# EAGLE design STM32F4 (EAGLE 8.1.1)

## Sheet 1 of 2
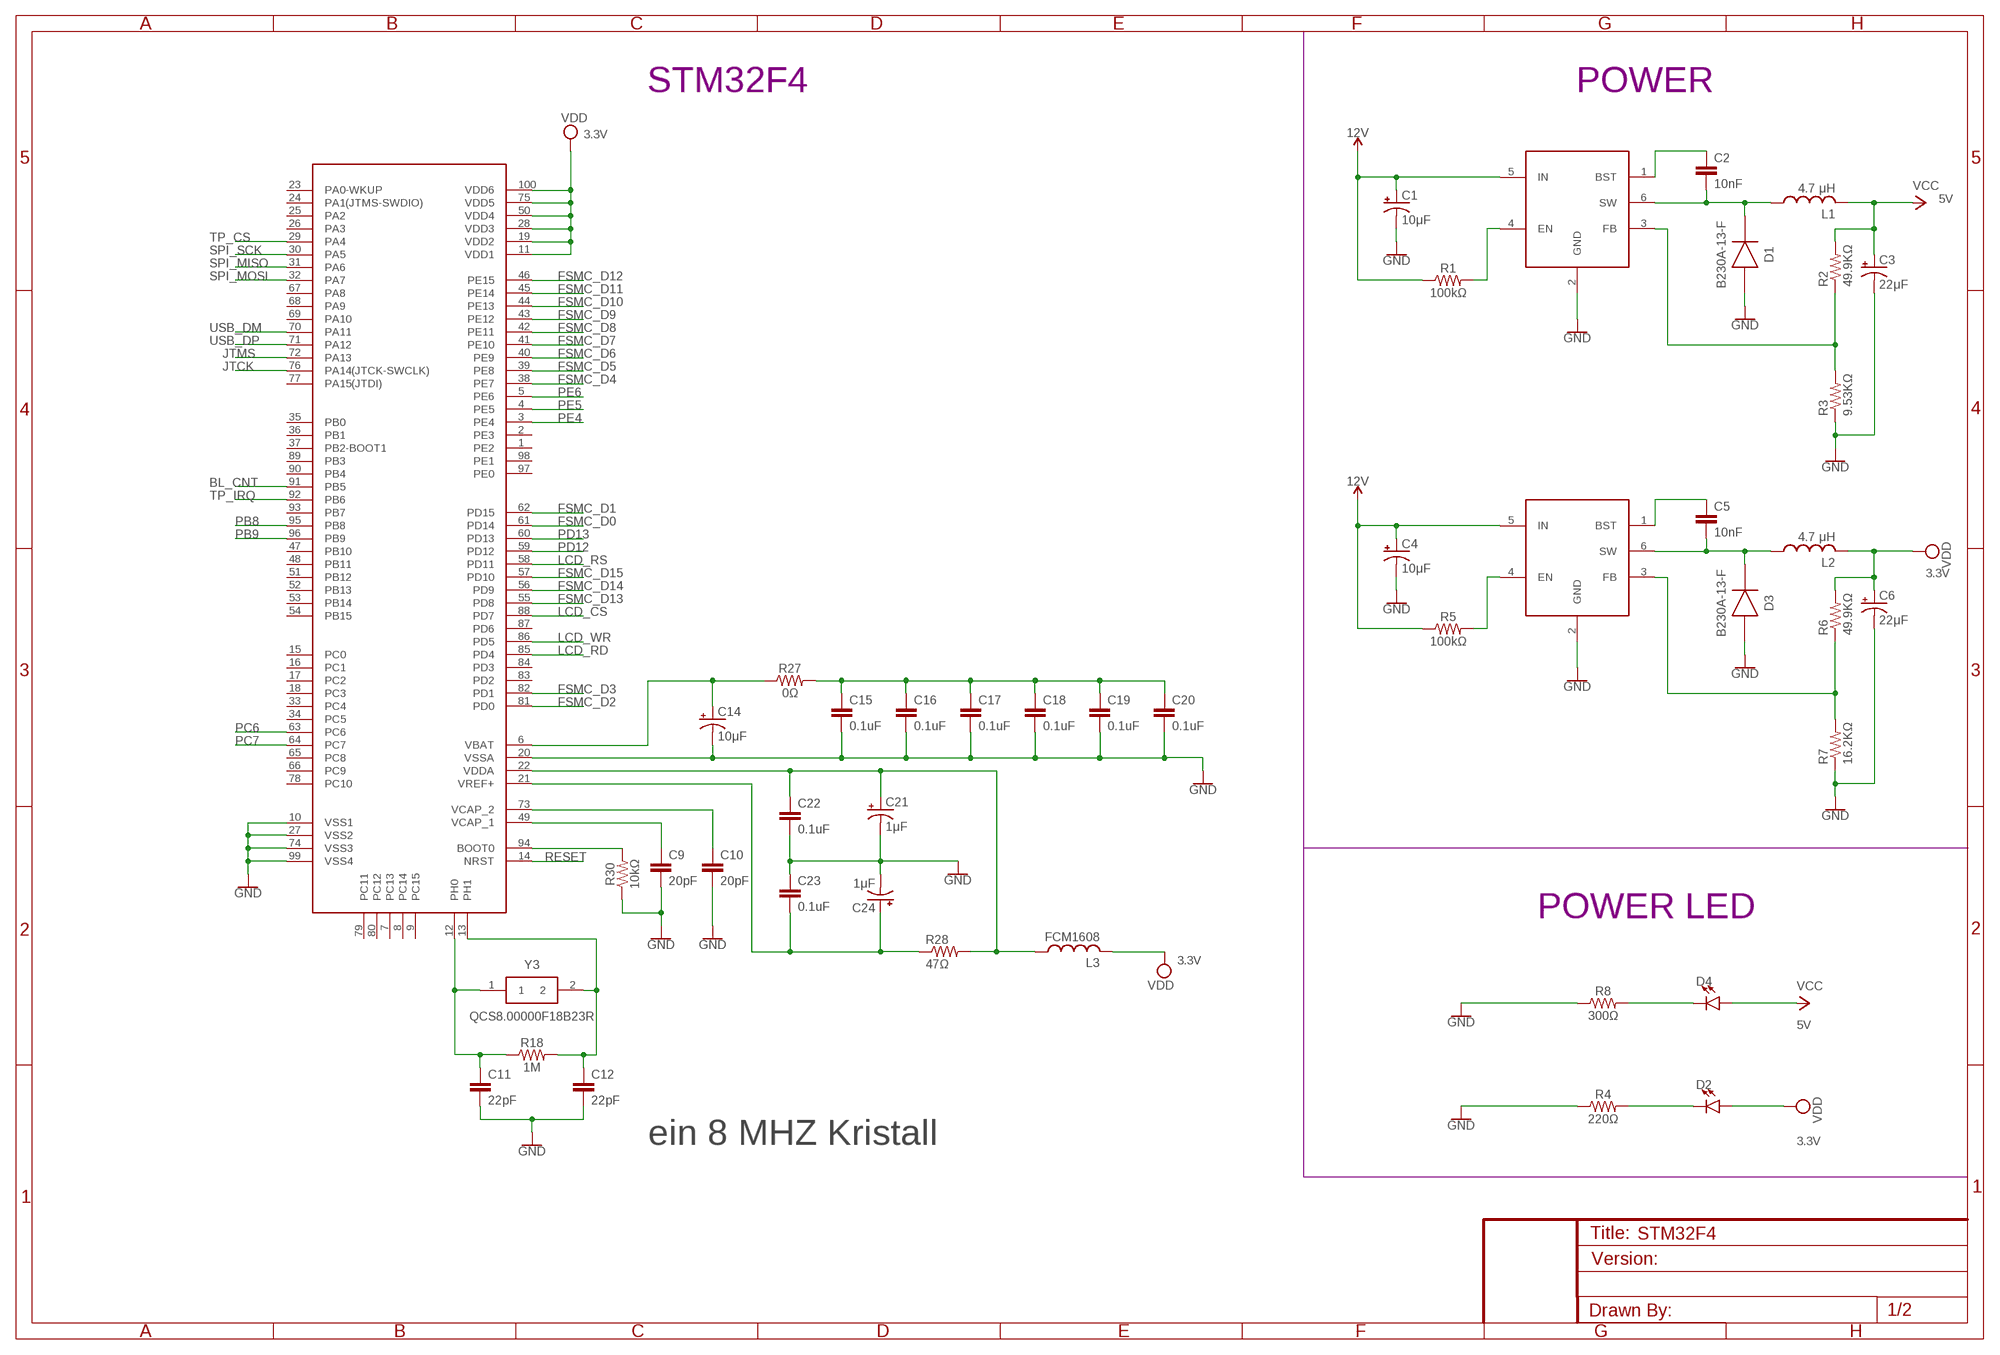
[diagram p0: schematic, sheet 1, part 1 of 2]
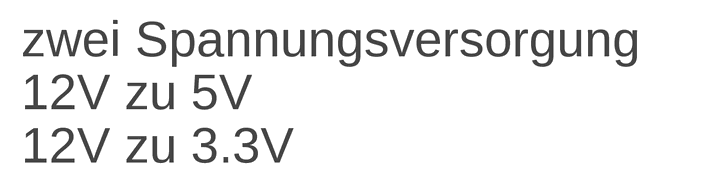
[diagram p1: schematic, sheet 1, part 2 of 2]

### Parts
C1  CAPACITOR_10UF  [E.CAPACITOR_10UF]
C2  10nF  10NF-0603-50V-10%  [0603]
C3  CAPACITOR_22UF  [E.CAPACITOR_10UF]
C4  CAPACITOR_10UF  [E.CAPACITOR_10UF]
C5  10nF  10NF-0603-50V-10%  [0603]
C6  CAPACITOR_22UF  [E.CAPACITOR_10UF]
C9  20pF  C-EUC0603  [C0603]
C10  20pF  C-EUC0603  [C0603]
C11  22pF  22PF-0603-50V-5%  [0603]
C12  22pF  22PF-0603-50V-5%  [0603]
C14  CAPACITOR_10UF  [E.CAPACITOR_10UF]
C15  0.1uF  0.1UF-0603-25V-5%  [0603]
C16  0.1uF  0.1UF-0603-25V-5%  [0603]
C17  0.1uF  0.1UF-0603-25V-5%  [0603]
C18  0.1uF  0.1UF-0603-25V-5%  [0603]
C19  0.1uF  0.1UF-0603-25V-5%  [0603]
C20  0.1uF  0.1UF-0603-25V-5%  [0603]
C21  CAPACITOR_1UF  [E.CAPACITOR_10UF]
C22  0.1uF  0.1UF-0603-25V-5%  [0603]
C23  0.1uF  0.1UF-0603-25V-5%  [0603]
C24  CAPACITOR_1UF  [E.CAPACITOR_10UF]
D1  B230A-13-F  [DIOM5226X230N]
D2  2  LED0603  [LED-0603]
D3  B230A-13-F  [DIOM5226X230N]
D4  1  LED0603  [LED-0603]
L1  A921CY-4R7M  [4.7μH]
L2  A921CY-4R7M  [4.7μH]
L3  FCM1608  [FCM1608]
R1  100kΩ  100KOHM-0603-1/10W-1%  [0603]
R2  49.9KΩ  R-US_R0603  [R0603]
R3  9.53KΩ  R-US_R0603  [R0603]
R4  220Ω  470OHM-0603-1/10W-1%  [0603]
R5  100kΩ  100KOHM-0603-1/10W-1%  [0603]
R6  49.9KΩ  R-US_R0603  [R0603]
R7  16.2KΩ  R-US_R0603  [R0603]
R8  300Ω  470OHM-0603-1/10W-1%  [0603]
R18  1M  1MOHM-0603-1/4W-5%  [0603]
R27  0Ω  0OHM-0603-1/10W-5%  [0603]
R28  47Ω  R-US_R0603  [R0603]
R30  10kΩ  10KOHM-0603-1/10W-1%  [0603]
U1  STM32F407VGT  [LQFP100_14X14]
U2  MP2359  [MP2359]
U3  MP2359  [MP2359]
Y3  QCS8.00000F18B23R  [QCS8.00000F18B23R]

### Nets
12V: C1.1(+) C4.1(+) R1.1 R5.1 U2.5(IN) U3.5(IN) ; also sheet 2
BL_CNT: U1.91(PB5) ; also sheet 2
FSMC_D0: U1.61(PD14) ; also sheet 2
FSMC_D1: U1.62(PD15) ; also sheet 2
FSMC_D2: U1.81(PD0) ; also sheet 2
FSMC_D3: U1.82(PD1) ; also sheet 2
FSMC_D4: U1.38(PE7) ; also sheet 2
FSMC_D5: U1.39(PE8) ; also sheet 2
FSMC_D6: U1.40(PE9) ; also sheet 2
FSMC_D7: U1.41(PE10) ; also sheet 2
FSMC_D8: U1.42(PE11) ; also sheet 2
FSMC_D9: U1.43(PE12) ; also sheet 2
FSMC_D10: U1.44(PE13) ; also sheet 2
FSMC_D11: U1.45(PE14) ; also sheet 2
FSMC_D12: U1.46(PE15) ; also sheet 2
FSMC_D13: U1.55(PD8) ; also sheet 2
FSMC_D14: U1.56(PD9) ; also sheet 2
FSMC_D15: U1.57(PD10) ; also sheet 2
GND: C1.2(-) C3.2(-) C4.2(-) C6.2(-) C9.2 C10.2 C11.2 C12.2 C14.2(-) C15.2 C16.2 C17.2 C18.2 C19.2 C20.2 C21.2(-) C22.2 C23.1 C24.2(-) D1.2(A) D3.2(A) R3.1 R4.1 R7.1 R8.1 R30.1 U1.10(VSS1) U1.20(VSSA) U1.27(VSS2) U1.74(VSS3) U1.99(VSS4) U2.2(GND) U3.2(GND) ; also sheet 2
JTCK: U1.76(PA14(JTCK-SWCLK)) ; also sheet 2
JTMS: U1.72(PA13) ; also sheet 2
LCD_CS: U1.88(PD7) ; also sheet 2
LCD_RD: U1.85(PD4) ; also sheet 2
LCD_RS: U1.58(PD11) ; also sheet 2
LCD_WR: U1.86(PD5) ; also sheet 2
N$1: R1.2 U2.4(EN)
N$2: C2.2 D1.1(K) L1.1 U2.6(SW)
N$3: C2.1 U2.1(BST)
N$4: D2.C R4.2
N$5: R2.1 R3.2 U2.3(FB)
N$6: R5.2 U3.4(EN)
N$7: C5.2 D3.1(K) L2.1 U3.6(SW)
N$8: C5.1 U3.1(BST)
N$9: R6.1 R7.2 U3.3(FB)
N$10: D4.C R8.2
N$17: C11.1 R18.1 U1.12(PH0) Y3.1
N$20: C12.1 R18.2 U1.13(PH1) Y3.2
N$21: C14.1(+) R27.1 U1.6(VBAT)
N$22: C9.1 U1.49(VCAP_1)
N$26: C10.1 U1.73(VCAP_2)
N$27: C15.1 C16.1 C17.1 C18.1 C19.1 C20.1 R27.2
N$28: R30.2 U1.94(BOOT0)
N$29: C23.2 C24.1(+) R28.1 U1.21(VREF+)
N$30: C21.1(+) C22.1 L3.1 R28.2 U1.22(VDDA)
PB8: U1.95(PB8) ; also sheet 2
PB9: U1.96(PB9) ; also sheet 2
PC6: U1.63(PC6) ; also sheet 2
PC7: U1.64(PC7) ; also sheet 2
PD12: U1.59(PD12) ; also sheet 2
PD13: U1.60(PD13) ; also sheet 2
PE4: U1.3(PE4) ; also sheet 2
PE5: U1.4(PE5) ; also sheet 2
PE6: U1.5(PE6) ; also sheet 2
RESET: U1.14(NRST) ; also sheet 2
SPI_MISO: U1.31(PA6) ; also sheet 2
SPI_MOSI: U1.32(PA7) ; also sheet 2
SPI_SCK: U1.30(PA5) ; also sheet 2
TP_CS: U1.29(PA4) ; also sheet 2
TP_IRQ: U1.92(PB6) ; also sheet 2
USB_DM: U1.70(PA11) ; also sheet 2
USB_DP: U1.71(PA12) ; also sheet 2
VCC: C3.1(+) D4.A L1.2 R2.2 ; also sheet 2
VDD: C6.1(+) D2.A L2.2 L3.2 R6.2 U1.11(VDD1) U1.19(VDD2) U1.28(VDD3) U1.50(VDD4) U1.75(VDD5) U1.100(VDD6) ; also sheet 2
Unconnected: U1.1(PE2) U1.2(PE3) U1.7(PC13) U1.8(PC14) U1.9(PC15) U1.15(PC0) U1.16(PC1) U1.17(PC2) U1.18(PC3) U1.23(PA0-WKUP) U1.24(PA1(JTMS-SWDIO)) U1.25(PA2) U1.26(PA3) U1.33(PC4) U1.34(PC5) U1.35(PB0) U1.36(PB1) U1.37(PB2-BOOT1) U1.47(PB10) U1.48(PB11) U1.51(PB12) U1.52(PB13) U1.53(PB14) U1.54(PB15) U1.65(PC8) U1.66(PC9) U1.67(PA8) U1.68(PA9) U1.69(PA10) U1.77(PA15(JTDI)) U1.78(PC10) U1.79(PC11) U1.80(PC12) U1.83(PD2) U1.84(PD3) U1.87(PD6) U1.89(PB3) U1.90(PB4) U1.93(PB7) U1.97(PE0) U1.98(PE1)

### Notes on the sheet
- STM32F4 | POWER
- 3.3V
- 5V
- zwei Spannungsversorgung
  12V zu 5V
  12V zu 3.3V
- 3.3V
- POWER LED
- 3.3V
- 5V
- ein 8 MHZ Kristall | 3.3V

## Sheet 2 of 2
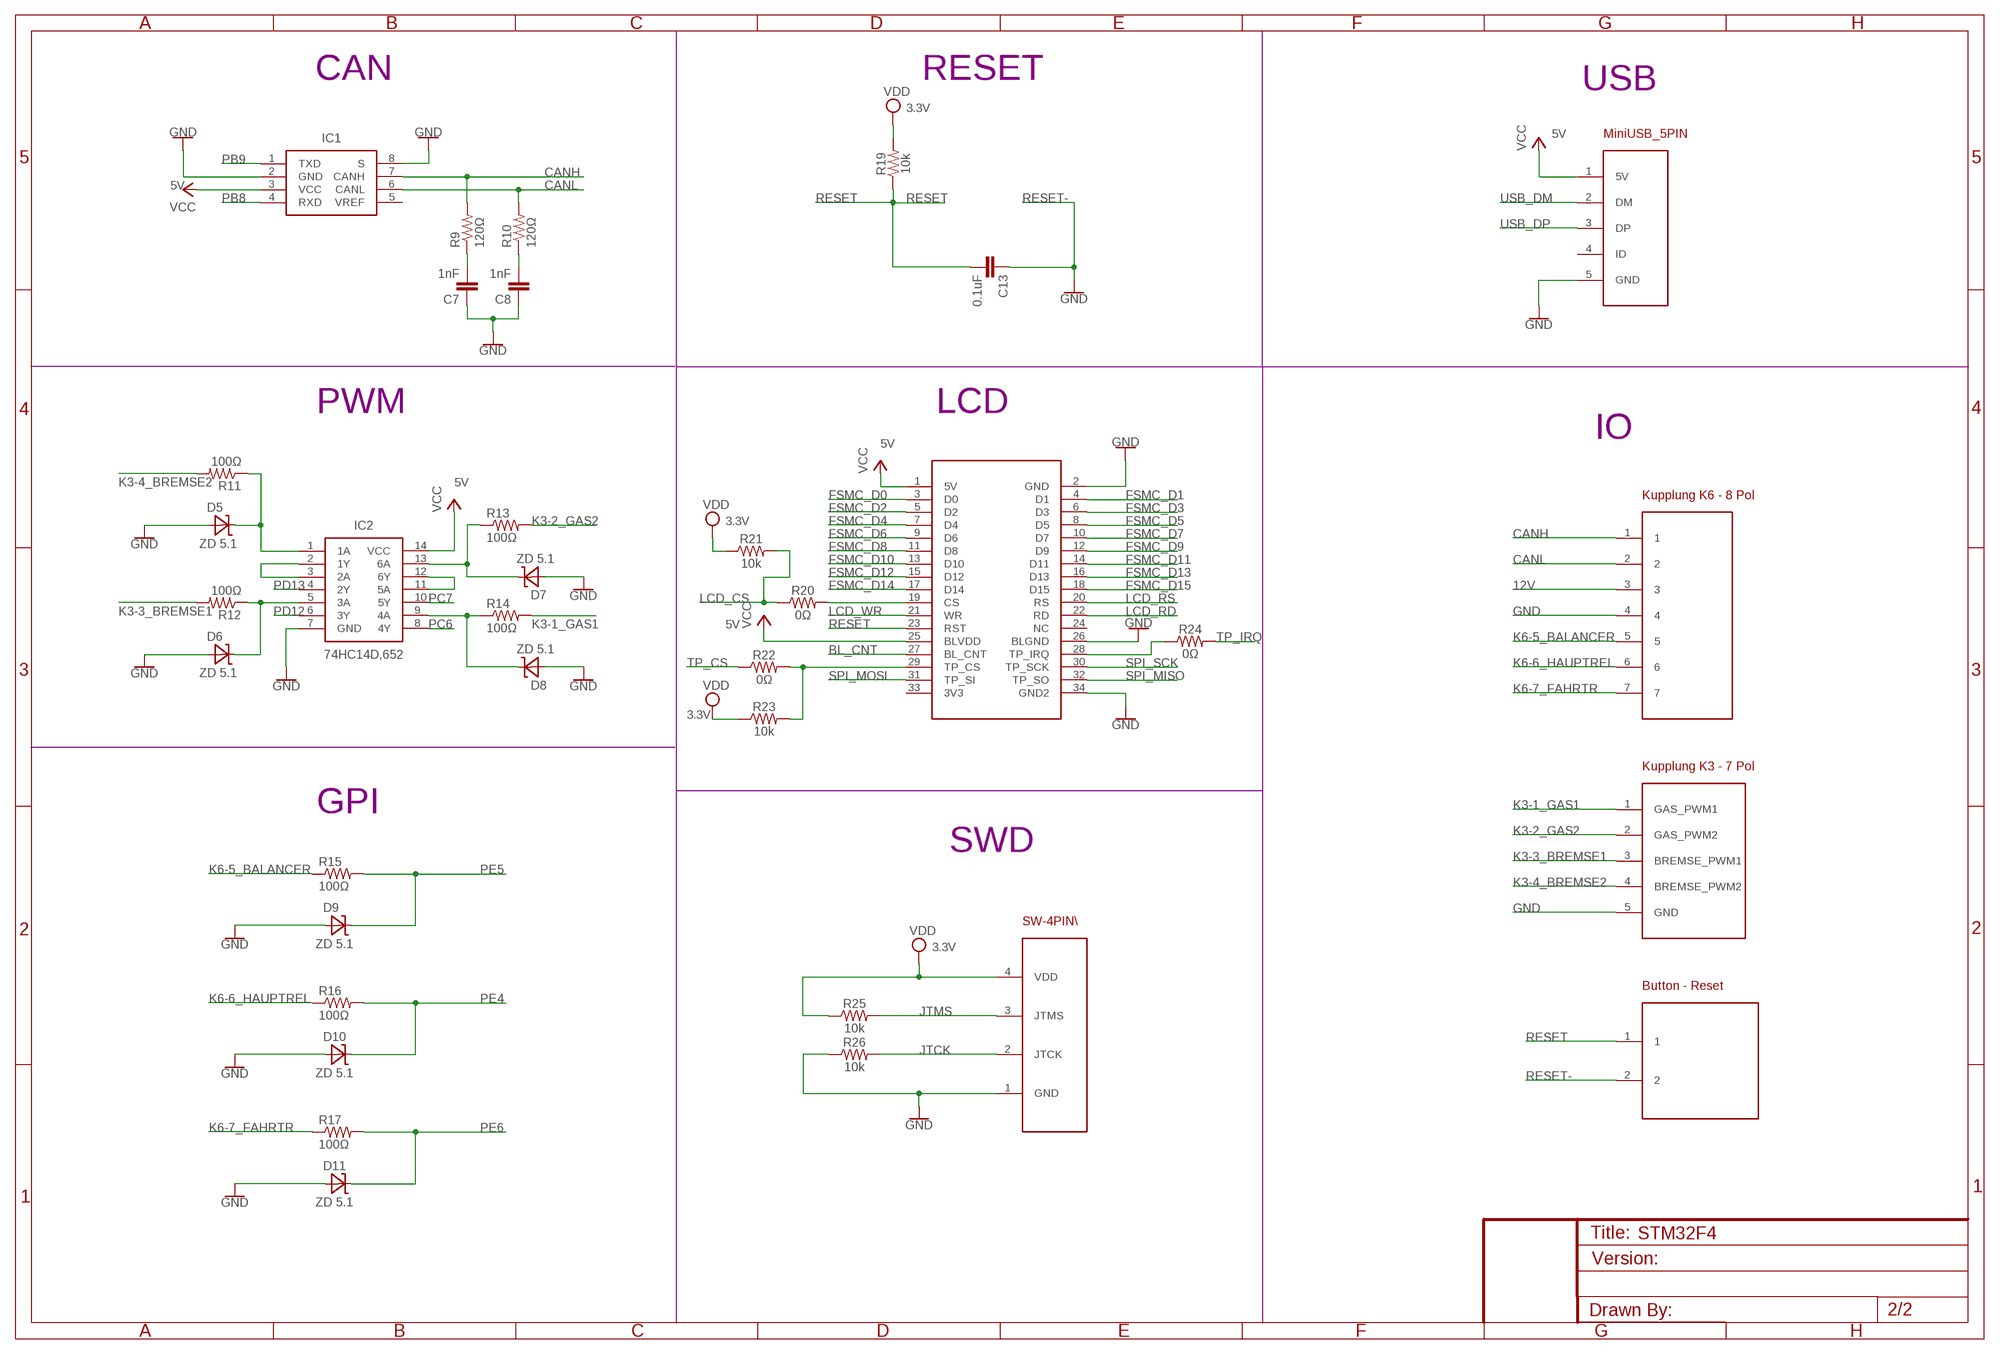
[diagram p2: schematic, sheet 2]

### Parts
C7  1nF  1.0NF/1000PF-0603-50V-10%  [0603]
C8  1nF  1.0NF/1000PF-0603-50V-10%  [0603]
C13  0.1uF  0.1UF-0603-25V-5%  [0603]
D5  ZD5.1V  [ZD5.1V]
D6  ZD5.1V  [ZD5.1V]
D7  ZD5.1V  [ZD5.1V]
D8  ZD5.1V  [ZD5.1V]
D9  ZD5.1V  [ZD5.1V]
D10  ZD5.1V  [ZD5.1V]
D11  ZD5.1V  [ZD5.1V]
IC1  TJA1050T_CM,118  [SOIC127P600X175-8N]
IC2  74HC14D,652  [SOIC127P600X175-14N]
R9  120Ω  R-US_R0603  [R0603]
R10  120Ω  R-US_R0603  [R0603]
R11  100Ω  R-US_R0603  [R0603]
R12  100Ω  R-US_R0603  [R0603]
R13  100Ω  R-US_R0603  [R0603]
R14  100Ω  R-US_R0603  [R0603]
R15  100Ω  R-US_R0603  [R0603]
R16  100Ω  R-US_R0603  [R0603]
R17  100Ω  R-US_R0603  [R0603]
R19  10k  10KOHM-0603-1/10W-1%  [0603]
R20  0Ω  0OHM-0603-1/10W-5%  [0603]
R21  10k  10KOHM-0603-1/10W-1%  [0603]
R22  0Ω  0OHM-0603-1/10W-5%  [0603]
R23  10k  10KOHM-0603-1/10W-1%  [0603]
R24  0Ω  0OHM-0603-1/10W-5%  [0603]
R25  10k  10KOHM-0603-1/10W-1%  [0603]
R26  10k  10KOHM-0603-1/10W-1%  [0603]
U$4  PIN34  [PIN34]
U$5  XH2.54  [XH2.54]
U$6  5PIN  [5PIN]
U$7  7PIN  [7PIN]
U$8  5-PIN  [5PIN]
U$9  2PIN  [2PIN]

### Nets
12V: U$7.3 ; also sheet 1
BL_CNT: U$4.27(BL_CNT) ; also sheet 1
CANH: IC1.7(CANH) R9.2 U$7.1
CANL: IC1.6(CANL) R10.2 U$7.2
FSMC_D0: U$4.3(D0) ; also sheet 1
FSMC_D1: U$4.4(D1) ; also sheet 1
FSMC_D2: U$4.5(D2) ; also sheet 1
FSMC_D3: U$4.6(D3) ; also sheet 1
FSMC_D4: U$4.7(D4) ; also sheet 1
FSMC_D5: U$4.8(D5) ; also sheet 1
FSMC_D6: U$4.9(D6) ; also sheet 1
FSMC_D7: U$4.10(D7) ; also sheet 1
FSMC_D8: U$4.11(D8) ; also sheet 1
FSMC_D9: U$4.12(D9) ; also sheet 1
FSMC_D10: U$4.13(D10) ; also sheet 1
FSMC_D11: U$4.14(D11) ; also sheet 1
FSMC_D12: U$4.15(D12) ; also sheet 1
FSMC_D13: U$4.16(D13) ; also sheet 1
FSMC_D14: U$4.17(D14) ; also sheet 1
FSMC_D15: U$4.18(D15) ; also sheet 1
GND: C7.1 C8.1 D5.1(A) D6.1(A) D7.1(A) D8.1(A) D9.1(A) D10.1(A) D11.1(A) IC1.2(GND) IC1.8(S) IC2.7(GND) R26.1 U$4.2(GND) U$4.26(BLGND) U$4.34(GND2) U$5.1(GND) U$6.5(GND) U$7.4 U$8.5(GND) ; also sheet 1
JTCK: R26.2 U$5.2(JTCK) ; also sheet 1
JTMS: R25.2 U$5.3(JTMS) ; also sheet 1
K3-1_GAS1: R14.2 U$8.1(GAS_PWM1)
K3-2_GAS2: R13.2 U$8.2(GAS_PWM2)
K3-3_BREMSE1: R12.2 U$8.3(BREMSE_PWM1)
K3-4_BREMSE2: R11.2 U$8.4(BREMSE_PWM2)
K6-5_BALANCER: R15.1 U$7.5
K6-6_HAUPTREL: R16.1 U$7.6
K6-7_FAHRTR: R17.1 U$7.7
LCD_CS: R20.1 R21.2 ; also sheet 1
LCD_RD: U$4.22(RD) ; also sheet 1
LCD_RS: U$4.20(RS) ; also sheet 1
LCD_WR: U$4.21(WR) ; also sheet 1
N$11: D5.2(C) IC2.1(1A) R11.1
N$12: IC2.2(1Y) IC2.3(2A)
N$13: C7.2 R9.1
N$14: C8.2 R10.1
N$15: D6.2(C) IC2.5(3A) R12.1
N$16: D8.2(C) IC2.9(4A) R14.1
N$18: IC2.11(5A) IC2.12(6Y)
N$19: D7.2(C) IC2.13(6A) R13.1
N$23: R20.2 U$4.19(CS)
N$24: R22.2 R23.2 U$4.29(TP_CS)
N$25: R24.1 U$4.28(TP_IRQ)
PB8: IC1.4(RXD) ; also sheet 1
PB9: IC1.1(TXD) ; also sheet 1
PC6: IC2.8(4Y) ; also sheet 1
PC7: IC2.10(5Y) ; also sheet 1
PD12: IC2.6(3Y) ; also sheet 1
PD13: IC2.4(2Y) ; also sheet 1
PE4: D10.2(C) R16.2 ; also sheet 1
PE5: D9.2(C) R15.2 ; also sheet 1
PE6: D11.2(C) R17.2 ; also sheet 1
RESET: C13.2 R19.1 U$4.23(RST) U$9.1 ; also sheet 1
RESET-: C13.1 U$9.2 ; supply symbol labelled GND
SPI_MISO: U$4.32(TP_SO) ; also sheet 1
SPI_MOSI: U$4.31(TP_SI) ; also sheet 1
SPI_SCK: U$4.30(TP_SCK) ; also sheet 1
TP_CS: R22.1 ; also sheet 1
TP_IRQ: R24.2 ; also sheet 1
USB_DM: U$6.2(DM) ; also sheet 1
USB_DP: U$6.3(DP) ; also sheet 1
VCC: IC1.3(VCC) IC2.14(VCC) U$4.1(5V) U$4.25(BLVDD) U$6.1(5V) ; also sheet 1
VDD: R19.2 R21.1 R23.1 R25.1 U$5.4(VDD) ; also sheet 1
Unconnected: IC1.5(VREF) U$4.24(NC) U$4.33(3V3) U$6.4(ID)

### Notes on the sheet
- CAN | RESET
- USB
- 3.3V
- 5V | MiniUSB_5PIN
- 5V
- PWM | LCD
- IO
- 5V
- 5V
- Kupplung K6 - 8 Pol
- 3.3V
- 5V
- 3.3V
- Kupplung K3 - 7 Pol
- GPI
- SWD
- SW-4PIN\
- 3.3V
- Button - Reset

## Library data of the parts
C1 C4 C14 = E.Capacitor_10uf:CAPACITOR_10UF
C2 C5 = SparkFun-Capacitors:10NF: 0.01uF/10nF/10,000pF ceramic capacitors; PROD_ID: CAP-00867
C3 C6 = E.Capacitor_10uf:CAPACITOR_22UF
C7 C8 = SparkFun-Capacitors:1.0NF/1000PF: 1nF/1,000pF ceramic capacitors; PROD_ID: CAP-07886
C9 C10 = rcl:C-EU: CAPACITOR, European symbol
C11 C12 = SparkFun-Capacitors:22PF: 22pF ceramic capacitors; PROD_ID: CAP-07876
C13 C15-C20 C22 C23 = SparkFun-Capacitors:0.1UF: 0.1µF ceramic capacitors; PROD_ID: CAP-08604
C21 C24 = E.Capacitor_10uf:CAPACITOR_1UF
D1 D3 = B230A-13-F:B230A-13-F: Schottky Diode 2A 30V 0.5Vf SMA Diodes Inc B230A-13-F, SMT Schottky Diode, 30V 2A, 2-Pin DO-214AC; DESCRIPTION: Schottky Diode 2A 30V 0.5Vf SMA Diodes Inc B230A-13-F, SMT Schottky Diode, 30V 2A, 2-Pin DO-214AC; HEIGHT: 2.3mm; MANUFACTURER_NAME: Diodes Inc.; MANUFACTURER_PART_NUMBER: B230A-13-F; RS_PART_NUMBER: 1219451; SUPPLIER_NAME: RS
D2 D4 = SparkFun-LED:LED: LED (Generic)
D5-D11 = ZD5.1V:ZD5.1V
IC1 = TJA1050T_CM,118:TJA1050T_CM,118: NXP - TJA1050T/CM,118 - CAN TRANSCEIVER, 1TX/RX, SOIC-8 Source: Datasheet; DESCRIPTION: NXP - TJA1050T/CM,118 - CAN TRANSCEIVER, 1TX/RX, SOIC-8; HEIGHT: 1.75mm; MANUFACTURER_NAME: NXP; MANUFACTURER_PART_NUMBER: TJA1050T/CM,118
IC2 = 74HC14D,652:74HC14D,652: 74HC14D,652, Hex Schmitt Trigger Inverter, HC, 5.2mA 2 to 6V 14-Pin SOIC Source: Datasheet; DESCRIPTION: 74HC14D,652, Hex Schmitt Trigger Inverter, HC, 5.2mA 2 to 6V 14-Pin SOIC; HEIGHT: 1.75mm; MANUFACTURER_NAME: NXP; MANUFACTURER_PART_NUMBER: 74HC14D,652; RS_PART_NUMBER: 1242255; SUPPLIER_NAME: RS
L1 L2 = A921CY-4R7M:A921CY-4R7M
L3 = FCM1608:FCM1608
R1 R5 = SparkFun-Resistors:100KOHM: 100kΩ resistor; PROD_ID: RES-07828; VALUE: 100k
R2 R3 R6 R7 = resistor:R-US_: RESISTOR, American symbol
R4 R8 = SparkFun-Resistors:470OHM: 470Ω resistor; PROD_ID: RES-07869; VALUE: 470
R9-R17 R28 = rcl:R-US_: RESISTOR, American symbol
R18 = SparkFun-Resistors:1MOHM: 1MΩ resistor; PROD_ID: RES-07868
R19 R21 R23 R25 R26 = SparkFun-Resistors:10KOHM: 10kΩ resistor; PROD_ID: RES-00824
R20 R22 R24 R27 = SparkFun-Resistors:0OHM: 0Ω resistor; PROD_ID: RES-08609; VALUE: 0
R30 = SparkFun-Resistors:10KOHM: 10kΩ resistor; PROD_ID: RES-00824; VALUE: 10k
U1 = stm32xx:STM32F407VGT
U2 U3 = MP2359:MP2359
U$4 = PIN_34:PIN34
U$5 = XH2.54:XH2.54
U$6 = XH2.54:5PIN
U$7 = XH2.54:7PIN
U$8 = XH2.54:5-PIN
U$9 = XH2.54:2PIN
Y3 = QCS8.00000F18B23R:QCS8.00000F18B23R: 8.000MHz QCS HC49/U-S SMD Crystal 8MHz, 20ppm, 2-Pin HC-49/U-S SMD; DESCRIPTION: 8.000MHz QCS HC49/U-S SMD Crystal 8MHz, 20ppm, 2-Pin HC-49/U-S SMD; HEIGHT: mm; MANUFACTURER_NAME: Qantek; MANUFACTURER_PART_NUMBER: QCS8.00000F18B23R; RS_PART_NUMBER: 8149507; SUPPLIER_NAME: RS

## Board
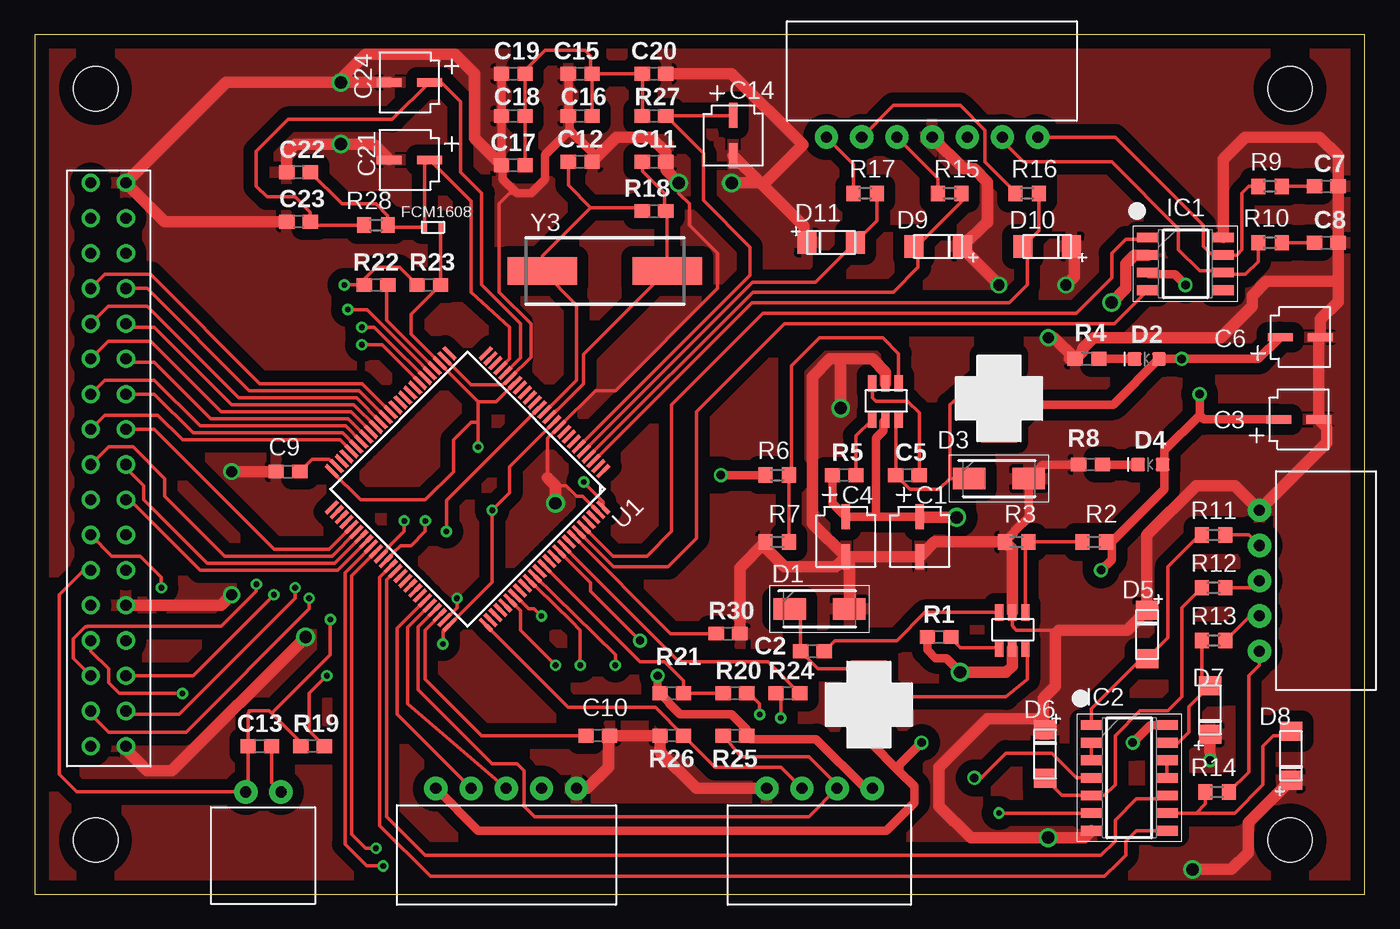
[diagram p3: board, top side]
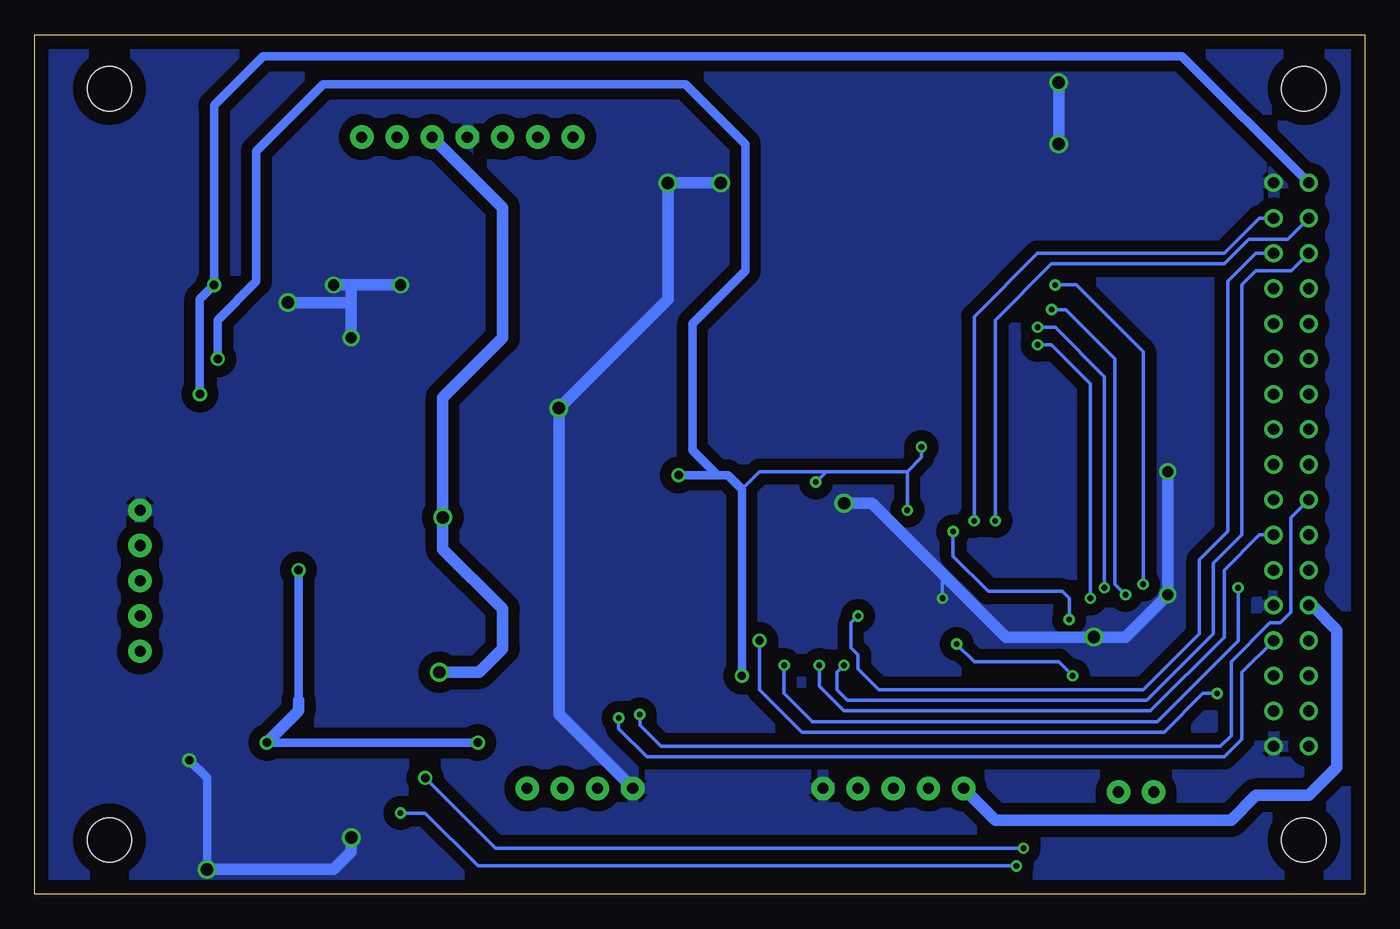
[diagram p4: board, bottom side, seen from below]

Size 96 x 62 mm. Coordinates in mm from the lower left corner, seen from the top.
Outline: 0,0 96,0 96,62 0,62 0,0
Copper layers (1*16): Top 0.035mm / dielectric 1.5mm / Bottom 0.035mm
Design rules "default": minimum track width 10mil, minimum drill 24mil, track to track 8mil, track to pad 8mil, pad to pad 8mil, via to via 8mil, smd to smd 8mil, copper to edge 40mil, drill to drill 8mil, minimum pad ring 10mil, minimum via ring 8mil, stop-mask expansion 4mil, vias tented up to drill 0mil, thermal gap 10mil
Holes 3.2 mm at 4.4,3.9 90.6,3.9 4.4,58.1 90.6,58.1

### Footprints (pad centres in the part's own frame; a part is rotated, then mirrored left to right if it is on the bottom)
E.CAPACITOR_10UF = smd 0.6 x 1.8: 1 2.15,3.6; 2 2.15,0.7
0603 = smd 1.1 x 1: 1 -0.85,0; 2 0.85,0
C0603 = smd 1.1 x 1: 1 -0.85,0; 2 0.85,0
DIOM5226X230N = smd 2.35 x 1.55: 1 -2.15,0; 2 2.15,0
LED-0603 = smd 1 x 1: A -0.877,0; C 0.877,0
ZD5.1V = smd 1.37 x 1.62: 1 0.1,-1; 2 3.6,-1
SOIC127P600X175-8N = smd 1.55 x 0.7: 1 -2.725,1.905; 2 -2.725,0.635; 3 -2.725,-0.635; 4 -2.725,-1.905; 5 2.725,-1.905; 6 2.725,-0.635; 7 2.725,0.635; 8 2.725,1.905
SOIC127P600X175-14N = smd 1.55 x 0.7: 1 -2.725,3.81; 2 -2.725,2.54; 3 -2.725,1.27; 4 -2.725,0; 5 -2.725,-1.27; 6 -2.725,-2.54; 7 -2.725,-3.81; 8 2.725,-3.81; 9 2.725,-2.54; 10 2.725,-1.27; 11 2.725,0; 12 2.725,1.27; 13 2.725,2.54; 14 2.725,3.81
4.7μH = smd 2.6 x 1.1: 1 0,-0.5; 2 0,-5.7
FCM1608 = smd 0.4 x 0.8: 1 0.2,-0.4; 2 1.4,-0.4
R0603 = smd 1 x 1.1: 1 -0.85,0; 2 0.85,0
LQFP100_14X14 = smd 1.2 x 0.28: 1 -7.85,6; 2 -7.85,5.5; 3 -7.85,5; 4 -7.85,4.5; 5 -7.85,4; 6 -7.85,3.5; 7 -7.85,3; 8 -7.85,2.5; 9 -7.85,2; 10 -7.85,1.5; 11 -7.85,1; 12 -7.85,0.5; 13 -7.85,0; 14 -7.85,-0.5; 15 -7.85,-1; 16 -7.85,-1.5; 17 -7.85,-2; 18 -7.85,-2.5; 19 -7.85,-3; 20 -7.85,-3.5; 21 -7.85,-4; 22 -7.85,-4.5; 23 -7.85,-5; 24 -7.85,-5.5; 25 -7.85,-6; 51 7.85,-6; 52 7.85,-5.5; 53 7.85,-5; 54 7.85,-4.5; 55 7.85,-4; 56 7.85,-3.5; 57 7.85,-3; 58 7.85,-2.5; 59 7.85,-2; 60 7.85,-1.5; 61 7.85,-1; 62 7.85,-0.5; 63 7.85,0; 64 7.85,0.5; 65 7.85,1; 66 7.85,1.5; 67 7.85,2; 68 7.85,2.5; 69 7.85,3; 70 7.85,3.5; 71 7.85,4; 72 7.85,4.5; 73 7.85,5; 74 7.85,5.5; 75 7.85,6 | smd 0.28 x 1.2: 26 -6,-7.85; 27 -5.5,-7.85; 28 -5,-7.85; 29 -4.5,-7.85; 30 -4,-7.85; 31 -3.5,-7.85; 32 -3,-7.85; 33 -2.5,-7.85; 34 -2,-7.85; 35 -1.5,-7.85; 36 -1,-7.85; 37 -0.5,-7.85; 38 0,-7.85; 39 0.5,-7.85; 40 1,-7.85; 41 1.5,-7.85; 42 2,-7.85; 43 2.5,-7.85; 44 3,-7.85; 45 3.5,-7.85; 46 4,-7.85; 47 4.5,-7.85; 48 5,-7.85; 49 5.5,-7.85; 50 6,-7.85; 76 6,7.85; 77 5.5,7.85; 78 5,7.85; 79 4.5,7.85; 80 4,7.85; 81 3.5,7.85; 82 3,7.85; 83 2.5,7.85; 84 2,7.85; 85 1.5,7.85; 86 1,7.85; 87 0.5,7.85; 88 0,7.85; 89 -0.5,7.85; 90 -1,7.85; 91 -1.5,7.85; 92 -2,7.85; 93 -2.5,7.85; 94 -3,7.85; 95 -3.5,7.85; 96 -4,7.85; 97 -4.5,7.85; 98 -5,7.85; 99 -5.5,7.85; 100 -6,7.85
MP2359 = smd 0.6 x 1.2: 1 0,0; 2 0.95,0; 3 1.9,0; 4 0,-2.6; 5 0.95,-2.6; 6 1.9,-2.6
PIN34 = drill 0.8: 1 0,0; 2 2.54,0; 3 0,-2.54; 4 2.54,-2.54; 5 0,-5.08; 6 2.54,-5.08; 7 0,-7.62; 8 2.54,-7.62; 9 0,-10.16; 10 2.54,-10.16; 11 0,-12.7; 12 2.54,-12.7; 13 0,-15.24; 14 2.54,-15.24; 15 0,-17.78; 16 2.54,-17.78; 17 0,-20.32; 18 2.54,-20.32; 19 0,-22.86; 20 2.54,-22.86; 21 0,-25.4; 22 2.54,-25.4; 23 0,-27.94; 24 2.54,-27.94; 25 0,-30.48; 26 2.54,-30.48; 27 0,-33.02; 28 2.54,-33.02; 29 0,-35.56; 30 2.54,-35.56; 31 0,-38.1; 32 2.54,-38.1; 33 0,-40.64; 34 2.54,-40.64
XH2.54 = drill 0.8 pad 1.676: 1 0,0; 2 2.54,0; 3 5.08,0; 4 7.62,0
5PIN = drill 0.8 pad 1.676: 1 3.81,0; 2 6.35,0; 3 8.89,0; 4 11.43,0; 5 13.97,0
7PIN = drill 0.8 pad 1.676: 1 3.81,1.27; 2 6.35,1.27; 3 8.89,1.27; 4 11.43,1.27; 5 13.97,1.27; 6 16.51,1.27; 7 19.05,1.27
2PIN = drill 0.8 pad 1.676: 1 3.81,0; 2 6.35,0
QCS8.00000F18B23R = smd 5 x 2: 1 -4.5,0; 2 4.5,0

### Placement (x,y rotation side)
C1  61.72,23.62 0 top
C2  56.13,17.53 180 top
C3  93.39,32.09 90 top
C4  56.39,23.62 0 top
C5  62.99,30.23 180 top
C6  93.49,38.02 90 top
C7  93.22,51.05 180 top
C8  93.22,46.99 180 top
C9  18.29,30.48 180 top
C10  40.64,11.43 0 top
C11  44.7,52.83 0 top
C12  39.37,52.83 0 top
C13  16.26,10.67 180 top
C14  48.26,52.58 0 top
C15  39.37,59.18 180 top
C16  39.37,56.13 180 top
C17  34.54,52.58 180 top
C18  34.54,56.13 180 top
C19  34.54,59.18 180 top
C20  44.7,59.18 0 top
C21  24.89,55.12 270 top
C22  19.05,52.07 180 top
C23  19.05,48.51 0 top
C24  24.89,60.71 270 top
D1  56.64,20.57 0 top
D2  80.26,38.61 180 top
D3  69.6,29.97 0 top
D4  80.52,30.99 180 top
D5  81.28,20.57 270 top
D6  73.91,11.94 270 top
D7  83.82,11.43 90 top
D8  89.66,8.13 90 top
D9  67.06,45.72 180 top
D10  74.93,45.72 180 top
D11  55.63,48.01 0 top
IC1  83.06,45.47 0 top
IC2  78.99,8.38 0 top
L1  60.2,16.76 0 top
L2  69.6,38.86 0 top
L3  27.94,48.51 0 top
R1  65.28,18.54 0 top
R2  76.45,25.4 0 top
R3  70.87,25.4 0 top
R4  75.95,38.61 0 top
R5  58.42,30.23 0 top
R6  53.59,30.23 180 top
R7  53.59,25.4 0 top
R8  76.2,30.99 0 top
R9  89.15,51.05 180 top
R10  89.15,46.99 180 top
R11  85.09,25.91 0 top
R12  85.09,22.1 0 top
R13  85.09,18.29 0 top
R14  85.34,7.37 0 top
R15  66.04,50.55 0 top
R16  71.63,50.55 0 top
R17  59.94,50.55 0 top
R18  44.7,49.28 180 top
R19  20.07,10.67 0 top
R20  50.55,14.48 0 top
R21  45.97,14.48 0 top
R22  24.64,43.94 180 top
R23  28.45,43.94 180 top
R24  54.36,14.48 0 top
R25  50.55,11.43 180 top
R26  45.97,11.43 0 top
R27  44.7,56.13 180 top
R28  24.64,48.26 0 top
R30  50.04,18.8 180 top
U1  31.24,29.21 225 top
U2  69.6,20.32 0 top
U3  60.45,36.83 0 top
U$4  4.05,51.31 0 top
U$5  52.83,7.62 0 top
U$6  25.15,7.62 0 top
U$7  76.2,55.88 180 top
U$8  88.39,13.72 90 top
U$9  11.43,7.37 0 top
Y3  41.15,44.96 180 top

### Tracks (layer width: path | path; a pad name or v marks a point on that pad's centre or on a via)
12V  (via drill 0.9 pad 1.27)
  Top 0.254: 57.32,29.97 R5.1
  Top 0.61: 60.71,27.22 C1.1 63.92,27.18 | 60.71,27.22 C4.1 57.57,28.19 R5.1 | U3.5 61.26,34.09 61.26,33.42 60.71,32.87 60.71,27.22 | R1.1 64.43,17.61 65.02,17.02 65.79,17.02 v66.8,16
  Top 0.813: U2.5 70.55,16.44 70.1,16 v66.8,16 | 63.92,27.18 v66.55,27.18
  Bottom 0.813: U$7.3 62.23,49.53 62.23,40.13 66.55,35.81 v66.55,27.18 66.55,24.89 62.23,20.57 62.23,17.71 63.94,16 v66.8,16
BL_CNT  (via drill 0.41 pad 0.81, 0.61 pad 1.02)
  Top 0.254: U$4.27 4.06,18.27 4.06,17.53 5.33,16.26 5.33,15.24 6.1,14.48 v10.67,14.48 | v43.69,18.29 40.13,21.84 40.13,22.44 U1.91
  Bottom 0.254: v43.69,18.29 43.69,14.73 40.64,11.68 14.48,11.68 11.68,14.48 v10.67,14.48
CANH
  Top 0.254: U$7.1 77.98,54.61 84.33,48.26 84.33,46.74 84.84,46.23 85.66,46.23 IC1.7 86.74,46.1 87.12,46.48 87.12,50.55 87.63,51.05 R9.2
CANL
  Top 0.254: U$7.2 69.85,54.36 71.37,52.83 77.72,52.83 82.55,48.01 82.55,46.48 84.07,44.96 85.66,44.96 IC1.6 85.91,44.7 87.38,44.7 88.3,45.63 R10.2
FSMC_D0  (via drill 0.41 pad 0.81)
  Top 0.254: U1.61 24.98,24.39 25.49,24.9 25.49,24.98 26.67,26.16 v26.67,26.92
  Bottom 0.254: U$4.3 5.57,47.24 8.38,47.24 10.16,45.47 22.61,45.47 26.67,41.4 v26.67,26.92
FSMC_D1  (via drill 0.41 pad 0.81)
  Top 0.254: U1.62 25.34,24.04 25.84,24.55 25.84,24.57 26.42,25.15 27.18,25.15 28.19,26.16 v28.19,26.92
  Bottom 0.254: U$4.4 7.62,48.77 10.16,46.23 23.62,46.23 28.19,41.66 v28.19,26.92
FSMC_D2  (via drill 0.41 pad 0.81)
  Top 0.254: 34.32,21.16 U1.81 35.05,20.45 35.05,19.05 v37.59,16.51
  Bottom 0.254: U$4.5 5.32,44.96 7.87,44.96 8.89,43.94 8.89,25.91 10.92,23.88 10.92,18.8 15.75,13.97 37.34,13.97 38.1,14.73 38.1,16 v37.59,16.51
FSMC_D3  (via drill 0.41 pad 0.81)
  Top 0.254: U1.82 34.7,21.54 35.65,20.59 36.05,20.59 v36.58,20.07
  Bottom 0.254: U$4.6 7.87,46.23 9.91,44.2 9.91,26.16 11.94,24.13 11.94,18.8 16,14.73 35.05,14.73 36.58,16.26 36.58,17.27 37.08,17.78 37.08,19.56 v36.58,20.07
FSMC_D4
  Top 0.254: U1.38 23.62,36.83 16.26,36.83 8.38,44.7 5.06,44.7 U$4.7
FSMC_D5
  Top 0.254: U1.39 23.42,36.32 15.49,36.32 8.13,43.69 U$4.8
FSMC_D6
  Top 0.254: U1.40 23.22,35.81 22.86,35.81 14.73,35.81 8.13,42.42 5.32,42.42 U$4.9
FSMC_D7
  Top 0.254: U1.41 23.02,35.31 14.22,35.31 8.64,40.89 6.84,40.89 U$4.10
FSMC_D8
  Top 0.254: U1.42 22.83,34.8 22.61,34.8 | 22.61,34.8 22.35,34.8 | 22.61,34.8 13.46,34.8 8.38,39.88 5.32,39.88 U$4.11
FSMC_D9
  Top 0.254: U1.43 22.63,34.29 12.7,34.29 8.64,38.35 6.84,38.35 U$4.12
FSMC_D10
  Top 0.254: U1.44 22.43,33.78 11.94,33.78 8.64,37.08 5.06,37.08 U$4.13
FSMC_D11
  Top 0.254: U1.45 22.23,33.27 11.43,33.27 8.64,36.07 U$4.14
FSMC_D12
  Top 0.254: U1.46 22.03,32.77 10.67,32.77 8.89,34.54 5.06,34.54 U$4.15
FSMC_D13
  Top 0.254: U1.55 21.27,24.89 17.27,24.89 8.64,33.53 U$4.16
FSMC_D14
  Top 0.254: U1.56 21.47,24.38 13.72,24.38 9.4,28.7 9.4,29.97 7.11,32.26 5.33,32.26 4.06,30.99 U$4.17
FSMC_D15
  Top 0.254: U1.57 21.66,23.88 12.45,23.88 7.87,28.45 7.87,29.46 6.59,30.75 U$4.18
GND  (via drill 0.41 pad 0.81, 0.61 pad 1.02, 0.8 pad 1.07, 0.9 pad 1.27)
  Top 0.254: 29.58,19.74 U1.74 30.48,20.67 v30.48,21.34 | U1.27 31.5,36.73 33.78,36.73 34.29,37.24 U1.20 35.81,38.73 35.81,41.15 33.53,43.43 33.53,49.78 34.29,50.55 34.8,50.55 | v46.48,51.31 46.48,50.55 47.24,49.78 47.24,48.26 49.28,46.23 49.28,43.69 41.91,36.32 40.48,36.32 U1.10 37.03,32.88 37.03,30.02 | IC1.2 80.21,45.97 | U2.2 70.55,19.37 70.87,19.05 73.91,19.05 74.17,19.05 | 37.59,29.46 38.35,29.46 39.12,28.7 39.53,28.7 U1.99
  Top 0.61: R8.1 72.76,30.99 D3.2 71.75,27.2 70.71,26.16 70.71,26.09 R3.1 | C19.2 C18.2 C17.2 33.78,52.49 33.78,51.56 34.8,50.55 35.81,50.55 36.83,51.56 36.83,53.34 38.61,55.12 | C15.2 C16.2 38.61,56.05 38.61,55.12 | 38.61,55.12 40.22,53.51 C12.2
  Top 0.813: C4.2 C1.2 64.95,25.4 R3.1 70.55,24.87 U2.2 | C4.2 58.79,24.07 D1.2 | U$6.5 39.88,7.62 41.4,9.14 41.4,11.34 C10.2 R26.1 45.12,10.25 47.75,7.62 U$5.1 | U$4.34 6.59,10.43 8.13,8.89 9.91,8.89 v19.56,18.54 | C22.2 18.2,53.51 18.8,54.1 v22.1,54.1 24.46,54.1 C21.2 | v22.1,58.56 13.84,58.56 U$4.2 9.38,48.51 C23.1 | C17.2 31.75,54.52 31.75,59.18 30.35,60.58 23.88,60.58 22.1,58.8 v22.1,58.56 | C12.2 42,54.61 44.45,54.61 45.55,53.51 C11.2 45.55,52.24 v46.48,51.31 | IC2.7 75.76,4.06 v73.15,4.06 67.56,4.06 65.28,6.35 65.28,9.14 68.77,12.64 72.62,12.64 72.81,12.45 | R30.1 50.89,23.54 R7.1 52.74,24.98 54.1,23.62 57.84,23.62 C4.2 | R4.1 75.64,39.15 75.64,39.36 76.41,40.13 85.6,40.13 87.88,42.42 87.88,43.18 88.9,44.2 94.07,44.2 | U3.2 61.4,37.66 60.45,38.61 57.91,38.61 | 57.91,38.61 57.4,38.61 56.13,37.34 56.13,26.73 C4.2 | C14.2 52.35,51.34 | U$7.4 67.06,52.32 67.82,52.32 68.77,51.37 68.77,48.44 68.67,48.44 D9.1 | 74.68,38.61 R4.1 | U$4.26 13.46,20.83 v14.22,21.59 | R4.1 73.57,40.13 v73.15,40.13 | C9.2 v14.22,30.48 | C20.2 50.29,59.18 55.43,54.04 52.73,51.34 52.35,51.34 | v83.57,1.78 86.36,1.78 87.58,3 87.58,5.15 D8.1 | C24.2 v22.1,58.56 | 37.03,30.02 37.59,29.46 v37.59,28.19 | 52.35,51.34 52.32,51.31 v50.29,51.31 | 57.91,38.61 58.17,38.35 v58.17,35.05 | v77.72,42.67 78.74,43.69 78.74,45.47 79.38,46.1 IC1.2 | IC1.8 85.78,53.02 87.38,54.61 92.71,54.61 94.07,53.25 C7.1 C8.1 94.07,44.2 | 94.07,44.2 94.07,42.74 92.79,41.47 C6.2 92.69,40.07 C3.2 93.25,33.68 93.25,32.55 U$8.5 86.61,29.46 83.82,29.46 80.26,25.91 80.28,25.89 D5.1 78.86,19.05 73.91,19.05 73.66,18.8 73.66,14.99 72.81,14.14 72.81,12.45
  Top 0.813: 52.35,51.34 55.53,48.16 55.53,47.01 D11.1 | v74.42,43.94 75.03,44.55 75.03,46.52 D10.1 | 67.16,46.38 D9.1 | D9.1 66.96,46.58 v69.6,43.94 | 72.81,12.45 72.81,11.94 D6.1 | D7.1 84.82,10.68 v84.84,9.65
  Bottom 0.254: v30.48,21.34 30.48,22.61 30.23,22.86
  Bottom 0.61: v84.84,9.65 83.57,8.38 v83.57,1.78
  Bottom 0.813: v14.22,30.48 v14.22,21.59 17.27,18.54 v19.56,18.54 25.91,18.54 30.23,22.86 35.56,28.19 v37.59,28.19 | v22.1,54.1 v22.1,58.56 | v46.48,51.31 v50.29,51.31 50.29,42.93 v58.17,35.05 58.17,12.95 U$5.1 | v74.42,43.94 72.9,43.94 | 72.9,43.94 v69.6,43.94 | 72.9,43.94 73.15,43.69 73.15,42.42 | 73.15,42.42 v73.15,40.13 | 73.15,42.42 73.41,42.67 v77.72,42.67 | v83.57,1.78 74.42,1.78 73.15,3.05 v73.15,4.06
  pour Bottom (isolate 0.813): 0,61.98 0,0 96.01,0 96.01,61.98
  pour Top (isolate 0.813): 0,61.98 0,0 96.01,0 96.01,61.98
JTCK
  Top 0.254: U$5.2 53.85,9.14 49.11,9.14 R26.2 44.79,13.46 39.37,13.46 38.51,13.46 U1.76
JTMS
  Top 0.254: R25.2 50.97,9.91 55.88,9.91 57.91,7.87 U$5.3 55.88,5.59 36.07,5.59 35.31,6.35 35.31,8.89 34.8,9.4 33.02,9.4 27.69,14.73 27.69,19.29 U1.72
K3-1_GAS1
  Top 0.254: 86.19,7.2 R14.2 87.63,8.8 87.63,15.75 88.39,16.51 U$8.1
K3-2_GAS2
  Top 0.254: R13.2 87.72,20.07 U$8.2
K3-3_BREMSE1
  Top 0.254: R12.2 87.88,22.1 U$8.3
K3-4_BREMSE2
  Top 0.254: U$8.4 87.63,25.91 R11.2
K6-5_BALANCER
  Top 0.254: U$7.5 65.19,51.65 R15.1
K6-6_HAUPTREL
  Top 0.254: U$7.6 61.98,56.9 66.8,56.9 68.58,55.12 68.58,52.83 70.78,50.63 R16.1
K6-7_FAHRTR
  Top 0.254: U$7.7 59.09,52.67 R17.1
LCD_CS
  Top 0.254: R20.1 R21.2 46.82,15.41 45.47,16.76 43.69,16.76 U1.88
LCD_RD  (via drill 0.41 pad 0.81)
  Top 0.254: U1.85 35.76,22.6 36.27,22.09 38.74,19.68 39.37,19.05 v39.37,16.51
  Bottom 0.254: U$4.22 7.62,25.91 10.16,23.37 10.16,18.54 15.49,13.21 37.59,13.21 39.37,14.99 v39.37,16.51
LCD_RS
  Top 0.254: U1.58 21.86,23.37 11.94,23.37 6.86,28.45 U$4.20
LCD_WR  (via drill 0.41 pad 0.81)
  Top 0.254: U1.86 41.91,17.27 v41.91,16.51 | U$4.21 5.57,24.38 7.62,24.38 9.14,22.86 v9.14,22.1
  Bottom 0.254: v9.14,22.1 9.14,18.29 14.99,12.45 39.88,12.45 41.91,14.48 v41.91,16.51
N$1
  Top 0.254: U2.4 69.54,17.78 66.8,17.78 66.13,18.45 R1.2
N$2
  Top 0.254: D1.1 55.28,19.78 C2.2 56.55,16.26 L1.1 | L1.1 | U2.6 71.63,17.6 71.63,15.49 70.1,14.22 62.23,14.22 L1.1
N$3
  Top 0.254: C2.1 57.75,18.29 62.23,18.29 64.26,20.32 U2.1
N$4
  Top 0.61: R4.2 D2.C
N$5
  Top 0.254: R2.1 R3.2 71.5,25.18 U2.3
N$6
  Top 0.254: U3.4 59.27,33.05 R5.2
N$7
  Top 0.254: 66.04,29.97 D3.1 | U3.6 62.14,34.02 C5.2 63.16,29.21 65.28,29.21 66.04,29.97 | L2.1 66.04,35.31 66.04,29.97
N$8
  Top 0.254: 63.5,30.57 C5.1 63.84,34.71 62.99,35.56 60.71,35.56 60.45,35.81 U3.1
N$9
  Top 0.254: 62.4,36.87 U3.3 | R7.2 R6.1 54.61,30.39 54.61,38.1 56.64,40.13 61.21,40.13 62.35,38.99 U3.3 | 62.35,37.47 U3.3
N$10
  Top 0.61: R8.2 D4.C
N$11
  Top 0.254: 76.27,12.36 IC2.1 76.27,13.36 79.88,16.97 D5.2 81.79,18.48 81.79,19.05 | 81.79,18.88 81.79,19.05 | 81.79,19.05 81.79,23.62 84.07,25.91 R11.1
N$12
  Top 0.254: IC2.3 IC2.2
N$13
  Top 0.254: R9.1 C7.2
N$14
  Top 0.254: R10.1 C8.2
N$15
  Top 0.254: R12.1 82.8,20.66 82.8,14.22 81.79,13.21 79.76,13.21 77.98,11.43 77.98,7.87 77.22,7.11 IC2.5 74.14,7.11 D6.2
N$16
  Top 0.254: IC2.9 83.82,5.84 | 83.82,5.84 84.49,6.52 R14.1 | 83.82,5.84 86.61,5.84 88.65,7.87 88.65,10.67 89.41,11.43 90.36,11.43 D8.2
N$17
  Top 0.254: U1.12 37.17,34.41 37.68,34.91 37.71,34.91 39.62,36.83 39.62,38.93 Y3.1 45.65,49.18 R18.1 45.47,49.36 45.47,50.55 43.85,52.16 C11.1
N$18
  Top 0.254: IC2.11 IC2.12
N$19
  Top 0.254: R13.1 84.24,15.41 84.62,15.03 D7.2 | D7.2 84.92,14.56 | IC2.13 82.55,10.92 83.31,11.68 83.31,13.52 D7.2
N$20
  Top 0.254: U1.13 39.12,37.08 39.12,42.49 Y3.2 36.65,46.05 40.13,49.53 | R18.2 43.6,49.53 40.13,49.53 | 40.13,49.53 38.52,51.14 C12.1
N$21
  Top 0.254: C14.1 50.37,56.13 R27.1 48.26,53.43 48.26,50.04 51.62,46.68 51.62,44.65 51.36,44.38 U1.6
N$22
  Top 0.254: U1.49 21.77,30.87 21.27,31.38 20.02,31.38 C9.1
N$23  (via drill 0.41 pad 0.81)
  Top 0.254: v52.32,12.95 52.32,13.72 51.56,14.48 R20.2
  Bottom 0.254: U$4.19 5.33,27.16 5.33,20.32 6.1,19.56 6.86,19.56 9.65,16.76 9.65,11.43 10.41,10.67 50.8,10.67 52.32,12.19 v52.32,12.95
N$24  (via drill 0.41 pad 0.81)
  Top 0.254: R23.2 26.33,45.21 24.64,45.21 23.79,44.36 R22.2 v22.35,43.94 | U$4.29 4.05,15.76 2.79,17.02 2.79,18.43 3.64,19.27 3.78,19.27 3.81,19.3 13.46,19.3 16,21.84 v16,22.35
  Bottom 0.254: v16,22.35 16,39.12 20.83,43.94 v22.35,43.94
N$25  (via drill 0.41 pad 0.81)
  Top 0.254: R24.1 53.85,14.14 v53.85,12.7
  Bottom 0.254: U$4.28 8.89,15.99 8.89,11.18 10.16,9.91 51.82,9.91 53.85,11.94 v53.85,12.7
N$26
  Top 0.254: C10.1 32.26,11.43 28.19,15.49 28.19,19.05 28.72,19.58 28.72,19.59 29.23,20.1 U1.73
N$27
  Top 0.254: R27.2 C20.1 C15.1 | C15.1 C16.1 | C15.1 40.13,59.27 40.13,60.45 39.73,60.86 36.83,60.86 35.39,59.42 C19.1 C18.1 C17.1
N$28
  Top 0.254: U1.94 45.9,18.8 R30.2
N$29
  Top 0.254: R28.1 20.15,48.26 C23.2 19.9,49.19 18.8,50.29 16.76,50.29 16,51.05 16,53.59 18.29,55.88 25.82,55.88 C24.1 29.33,58.56 30.73,57.15 30.73,52.07 32.26,50.55 32.26,43.94 35.05,41.15 35.05,38.68 U1.21
N$30
  Top 0.254: C22.1 22.19,49.78 24.64,49.78 25.49,48.93 R28.2 25.63,48.11 L3.1 28.14,52.62 C21.1 31.5,49.96 31.5,43.43 34.29,40.89 34.29,38.62 U1.22
PB8
  Top 0.254: IC1.4 77.92,41.15 54.1,41.15 47.75,34.8 47.75,25.65 45.72,23.62 41.78,23.62 U1.95
PB9
  Top 0.254: IC1.1 80.21,47.24 78.74,47.24 77.72,46.23 77.72,44.45 75.18,41.91 52.58,41.91 45.97,35.31 45.97,26.16 44.2,24.38 41.73,24.38 U1.96
PC6
  Top 0.254: IC2.8 79.5,4.57 78.74,3.81 78.74,2.79 78.23,2.29 | 78.23,2.29 77.98,2.03 | 25.69,23.63 U1.63 24.89,22.86 24.89,5.33 24.89,4.94 28.56,1.27 77.22,1.27 78.23,2.29
PC7
  Top 0.254: IC2.10 81.47,6.86 79.5,6.86 77.98,5.33 77.98,3.81 76.96,2.79 28.19,2.79 25.4,5.59 25.4,22.66 U1.64
PD12  (via drill 0.41 pad 0.81)
  Top 0.254: U1.59 24.28,25.05 22.4,23.17 22.4,3.6 23.97,2.03 v25.15,2.03 | IC2.6 v69.6,5.84
  Bottom 0.254: v25.15,2.03 64.01,2.03 67.82,5.84 v69.6,5.84
PD13  (via drill 0.41 pad 0.81, 0.61 pad 1.02)
  Top 0.254: 24.63,24.69 U1.60 22.86,22.95 22.86,4.32 23.88,3.3 v24.64,3.3 | IC2.4 75.18,8.38 73.41,10.16 70.1,10.16 68.33,8.38 v67.82,8.38
  Bottom 0.254: v67.82,8.38 62.74,3.3 v24.64,3.3
PE4
  Top 0.254: U1.3 51.77,42.67 70.36,42.67 71.63,43.94 71.63,46.42 D10.2 72.48,47.87 R16.2
PE5
  Top 0.254: U1.4 51.83,43.43 61.98,43.43 63.76,45.21 63.76,46.42 D9.2 63.66,46.72 66.89,49.95 R15.2 66.55,50.2
PE6
  Top 0.254: 60.83,50.51 R17.2 60.79,48.57 D11.2 56.35,44.13 51.82,44.13 U1.5
RESET  (via drill 0.41 pad 0.81)
  Top 0.254: R19.1 19.22,10.92 17.1,13.04 | 17.1,13.04 16.93,13.21 15.57,13.21 | 15.49,13.21 15.57,13.21 | 15.57,13.21 15.41,13.04 C13.2 15.41,7.53 U$9.1 3.05,7.37 1.78,8.64 1.78,21.59 3.56,23.37 U$4.23 | 17.1,13.04 21.34,17.27 v21.34,19.81 | v29.72,26.16 29.72,28.39 U1.14
  Bottom 0.254: v29.72,26.16 29.72,24.38 27.18,21.84 21.84,21.84 21.34,21.34 v21.34,19.81
RESET-
  Top 0.254: C13.1 17.11,8.04 U$9.2
SPI_MISO  (via drill 0.41 pad 0.81)
  Top 0.254: U1.31 25.47,39.93 25.46,39.93 24.5,40.89 v23.62,40.89 | U$4.32 6.84,12.95 10.41,12.95 18.8,21.34 v18.8,22.1
  Bottom 0.254: v23.62,40.89 22.35,40.89 18.8,37.34 v18.8,22.1
SPI_MOSI  (via drill 0.41 pad 0.81)
  Top 0.254: U1.32 25.07,39.62 v23.62,39.62 | U$4.31 4.05,12.97 5.33,11.68 10.92,11.68 19.81,20.57 v19.81,21.34
  Bottom 0.254: v19.81,21.34 19.81,36.83 22.61,39.62 v23.62,39.62
SPI_SCK  (via drill 0.41 pad 0.81)
  Top 0.254: U1.30 28.52,37.62 28.01,38.12 28.01,38.14 23.99,42.16 v22.61,42.16 | v17.27,21.59 11.43,15.75 U$4.30
  Bottom 0.254: v22.61,42.16 21.59,42.16 18.03,38.61 18.03,22.35 v17.27,21.59
TP_CS
  Top 0.254: R22.1 25.4,43.85 25.4,41.4 U1.29
TP_IRQ
  Top 0.254: R24.2 52.92,16.76 46.52,16.76 U1.92
USB_DM
  Top 0.254: U$6.2 26.16,12.95 26.16,18.8 26.16,19.18 U1.70 28.14,21.18
USB_DP
  Top 0.254: U$6.3 26.92,13.72 26.92,19.23 U1.71 28.52,20.8
VCC  (via drill 0.61 pad 1.02)
  Top 0.61: D4.A 81.53,30.85 | 81.53,30.85 81.53,29.21 77.72,25.4 | R2.2 77.72,25.4 | 62.43,8.83 63.5,7.76 63.5,6.6 61.47,4.57 32,4.57 U$6.1 | 62.43,8.83 L1.2 | IC2.14 80.52,12.19 v79.25,10.92 | 62.43,8.83 62.43,9.34 v64.01,10.92 | 77.72,25.4 77.72,24.13 v76.96,23.37 | 81.53,30.85 81.53,32 84.07,34.54 | 84.07,34.54 v84.07,36.07 | v83.06,43.94 82.3,44.7 80.46,44.7 IC1.3 | C3.1 84.38,34.24 84.07,34.54
  Bottom 0.61: v79.25,10.92 v64.01,10.92 | v76.96,23.37 76.96,13.97 | v84.07,36.07 84.07,42.93 v83.06,43.94 83.06,56.9 79.5,60.45 13.19,60.45 U$4.1
  Bottom 0.813: U$4.25 3.81,20.83 2.03,19.05 2.03,9.14 4.06,7.11 7.87,7.11 9.65,5.33 26.67,5.33 U$6.1 | 76.96,13.97 76.96,13.21 v79.25,10.92
VDD  (via drill 0.41 pad 0.81, 0.61 pad 1.02)
  Top 0.254: L3.2 29.3,48.07 R23.1 27.18,41.82 27.18,40.39 28.72,38.84 28.72,38.83 29.23,38.32 U1.28 32,35.52 | 37.5,34.03 U1.11 34.29,30.84 34.29,28.96 v33.02,27.69 33.02,22.5 U1.75 29.46,18.95 v29.46,18.03 | U1.50 23.52,28.45 28.19,28.45 30.23,30.48 30.23,32.77 31.5,34.04 32,34.04 | v39.62,29.72 41.03,28.31 U1.100 | 32,34.04 32,35.52 | 32,34.04 v32,32.26 | 32,35.52 33.31,35.52 U1.19 | R19.2 19.81,11.77 19.81,14.48 v21.08,15.75
  Top 0.61: 81.26,38.73 D2.A | U$5.4 59.94,7.62 56.39,11.18 51.65,11.18 R25.1 51.4,11.85 50.29,12.95 46.58,12.95 45.77,13.77 45.77,13.84 R21.1 44.96,14.64 v44.96,15.75 | L2.2 71.74,35.31 77.84,35.31 D2.A | v49.53,30.23 R6.2 | D2.A v82.79,38.61 88.32,38.61 C6.1
  Bottom 0.254: 44.96,29.21 43.69,30.48 38.86,30.48 | 33.02,30.48 32,31.5 v32,32.26 | 33.02,30.48 38.86,30.48 | v33.02,27.69 33.02,30.48 | v29.46,18.03 28.19,16.76 22.1,16.76 v21.08,15.75 | 38.86,30.48 v39.62,29.72
  Bottom 0.61: 46.74,30.23 45.97,30.23 44.96,29.21 v44.96,15.75 | 46.74,30.23 v49.53,30.23 | 46.74,30.23 48.51,32 48.51,41.15 44.7,44.96 44.7,54.1 49.02,58.42 75.18,58.42 80.01,53.59 80.01,44.2 82.8,41.4 82.79,41.39 v82.79,38.61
